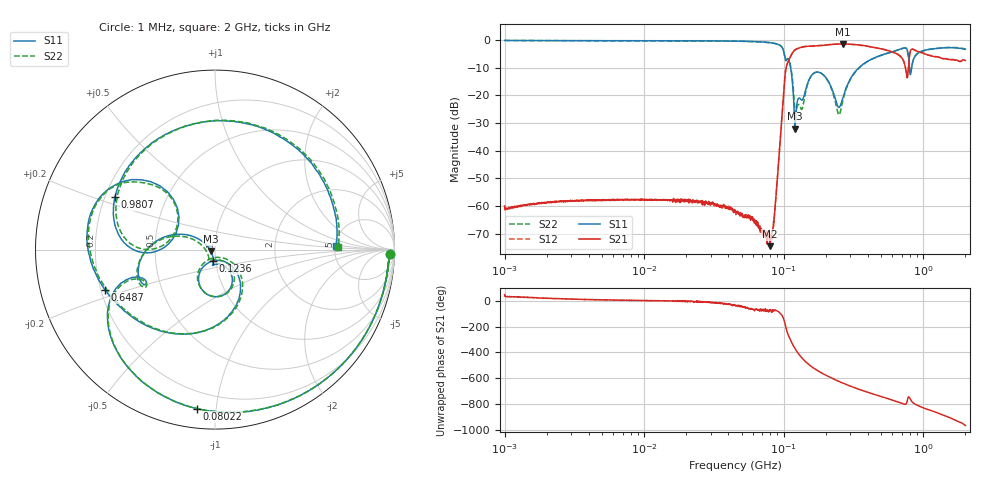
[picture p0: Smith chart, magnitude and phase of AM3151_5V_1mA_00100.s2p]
! Date/Time: Fri Jun 26 10:31:43 2020
! Network Analyzer:  Rev:
! Sweep from 1000000.0 to 2000000000.0, 1601 Points ! Power Supply: 0 V, 0 A
# HZ S DB R 50
!freq MagS11 AngS11 MagS21 AngS21 MagS12 AngS12 MagS22 AngS22
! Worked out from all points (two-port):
!   1601 points, 1 MHz to 2 GHz, reference 50 ohm
!   highest |S21| = -1.43 dB at 265.6 MHz (marker M1); lowest = -74.5 dB at 79.46 MHz (marker M2)
!   |S21| within 3 dB of the highest: 116.1 MHz to 603.1 MHz (487 MHz wide, 135 % of centre); 803.2 MHz to 953 MHz (149.8 MHz wide, 17.1 % of centre)
!   lowest |S11| = -32.0 dB at 120.1 MHz (marker M3), VSWR 1.05, Z = 47.7 - j0.818 ohm
!   |S11| at or under -10 dB: 111.9 MHz to 346.2 MHz (234.3 MHz wide, 102 % of centre); 795.4 MHz to 824 MHz (28.61 MHz wide, 3.53 % of centre)
!   |S22| runs from -27.1 to -0.2 dB; largest |S21 - S12| = 0.0095
!   S11 on the Smith chart (normalised r, x): 1 MHz: 36, -44; 80.22 MHz: 0.10, -0.89; 123.6 MHz: 0.97, -0.13; 648.7 MHz: 0.22, -0.17; 980.7 MHz: 0.24, +0.23; 2 GHz: 5.13, +0.42
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1000000  -0.19 -1.6  -59.95 50.8  -61.29 38.0  -0.19 -1.5
3555161  -0.27 -3.9  -58.08 12.3  -58.25 13.6  -0.26 -3.9
1.263916e7  -0.29 -12.8  -57.78 3.0  -57.81 2.7  -0.29 -12.8
4.493426e7  -0.43 -47.0  -61.62 -37.0  -62.47 -34.5  -0.43 -47.0
7.946115e7  -0.97 -95.1  -74.50 -76.3  -70.95 -74.6  -0.97 -95.1
8.021973e7  -0.98 -96.5  -71.45 -72.0  -70.46 -70.8  -1.01 -96.5
8.533003e7  -1.22 -107.1  -63.97 -75.8  -64.92 -69.7  -1.22 -106.9
1.031876e8  -7.45 -156.6  -10.82 161.9  -10.80 161.9  -7.38 -155.0
1.10809e8  -8.89 176.4  -6.37 65.1  -6.38 65.2  -8.53 179.3
1.20129e8  -32.04 -160.0  -3.65 -8.6  -3.66 -8.6  -25.30 178.7
1.236025e8  -23.75 -98.3  -3.27 -29.7  -3.26 -29.7  -24.95 -127.6
1.378729e8  -21.11 -70.3  -2.50 -93.2  -2.48 -93.1  -23.29 -60.9
1.589914e8  -12.64 -68.7  -2.20 -151.9  -2.20 -152.0  -12.69 -66.3
1.941001e8  -12.81 -109.9  -1.90 150.4  -1.90 150.6  -12.89 -111.1
2.655783e8  -20.69 -49.1  -1.43 81.3  -1.44 81.2  -21.72 -39.8
3.756664e8  -8.56 -77.8  -2.06 19.9  -2.09 19.7  -8.64 -76.0
5.652395e8  -4.65 -137.8  -3.96 -41.3  -3.94 -41.3  -4.71 -138.4
6.487302e8  -3.70 -159.9  -5.06 -61.8  -5.09 -62.0  -3.77 -161.5
8.148812e8  -11.71 172.8  -3.57 -51.6  -3.57 -51.6  -11.54 170.0
9.807482e8  -4.01 152.1  -4.62 -107.1  -4.62 -106.8  -4.05 149.0
1.4274e9  -2.83 81.6  -6.76 -171.8  -6.72 -171.7  -2.77 78.4
2e9  -3.40 1.9  -7.43 112.3  -7.57 111.7  -3.25 1.4
